FUNCTION_BLOCK FB_LN_IED_LD1_LLN0 EXTENDS FB_AcsiCommonLogicalNodeClass
VAR_INPUT
	NamPlt: FB_DO_IED_LD1_LLN0_NamPlt := (sClass:='LPL', bLinkResult:=THIS^.AddDataToContainer(ipData:=NamPlt));
	Beh: FB_DO_IED_LD1_LLN0_Beh := (sClass:='ENS', bLinkResult:=THIS^.AddDataToContainer(ipData:=Beh));
	Health: FB_DO_IED_LD1_LLN0_Health := (sClass:='ENS', bLinkResult:=THIS^.AddDataToContainer(ipData:=Health));
	Mod_: FB_DO_IED_LD1_LLN0_Mod := (sObjectName:='Mod', sClass:='ENC', bLinkResult:=THIS^.AddDataToContainer(ipData:=Mod_));
	
	DS1: FB_DS_IED_LD1_LLN0_DS1 := (bLinkResult:=THIS^.AddDataSetToContainer(ipDataSet:=DS1));
	DS2: FB_DS_IED_LD1_LLN0_DS2 := (bLinkResult:=THIS^.AddDataSetToContainer(ipDataSet:=DS2));
	DS3: FB_DS_IED_LD1_LLN0_DS3 := (bLinkResult:=THIS^.AddDataSetToContainer(ipDataSet:=DS3));
	DS4: FB_DS_IED_LD1_LLN0_DS4 := (bLinkResult:=THIS^.AddDataSetToContainer(ipDataSet:=DS4));
	DS5: FB_DS_IED_LD1_LLN0_DS5 := (bLinkResult:=THIS^.AddDataSetToContainer(ipDataSet:=DS5));
	DS6: FB_DS_IED_LD1_LLN0_DS6 := (bLinkResult:=THIS^.AddDataSetToContainer(ipDataSet:=DS6));
	DS7: FB_DS_IED_LD1_LLN0_DS7 := (bLinkResult:=THIS^.AddDataSetToContainer(ipDataSet:=DS7));
	DS8: FB_DS_IED_LD1_LLN0_DS8 := (bLinkResult:=THIS^.AddDataSetToContainer(ipDataSet:=DS8));
	
	urcb101: FB_ScsmUrCBImplClass := (RptID:=(sValue:='IEDLD1/LLN0.urcb101'), DatSet:=(sValue:='IEDLD1/LLN0.DS1'), ConfRev:=(nValue:=1), OptFlds:=(SequenceNumber:=TRUE, ReportTimeStamp:=TRUE, ReasonForInclusion:=TRUE, DataSetName:=TRUE, DataReference:=FALSE, BufferOverflow:=FALSE, EntryID:=FALSE, ConfRevision:=TRUE), TrgOps:=(DataChange:=TRUE, QualityChange:=TRUE, DataUpdate:=TRUE, Integrity:=TRUE, GeneralInterrogation:=TRUE), IntgPd:=(nValue:=5000), bLinkResult:=THIS^.AddUnbufferedReportControlBlockToContainer(ipUnbufferedReportControlBlock:=urcb101));
	brcb101: FB_ScsmBrCBImplClass := (RptID:=(sValue:='IEDLD1/LLN0.brcb101'), DatSet:=(sValue:='IEDLD1/LLN0.DS1'), ConfRev:=(nValue:=1), OptFlds:=(SequenceNumber:=TRUE, ReportTimeStamp:=TRUE, ReasonForInclusion:=TRUE, DataSetName:=TRUE, DataReference:=FALSE, BufferOverflow:=TRUE, EntryID:=TRUE, ConfRevision:=TRUE), TrgOps:=(DataChange:=TRUE, QualityChange:=TRUE, DataUpdate:=TRUE, Integrity:=TRUE, GeneralInterrogation:=TRUE), IntgPd:=(nValue:=5000), bLinkResult:=THIS^.AddBufferedReportControlBlockToContainer(ipBufferedReportControlBlock:=brcb101));
END_VAR
VAR
END_VAR

END_FUNCTION_BLOCK
